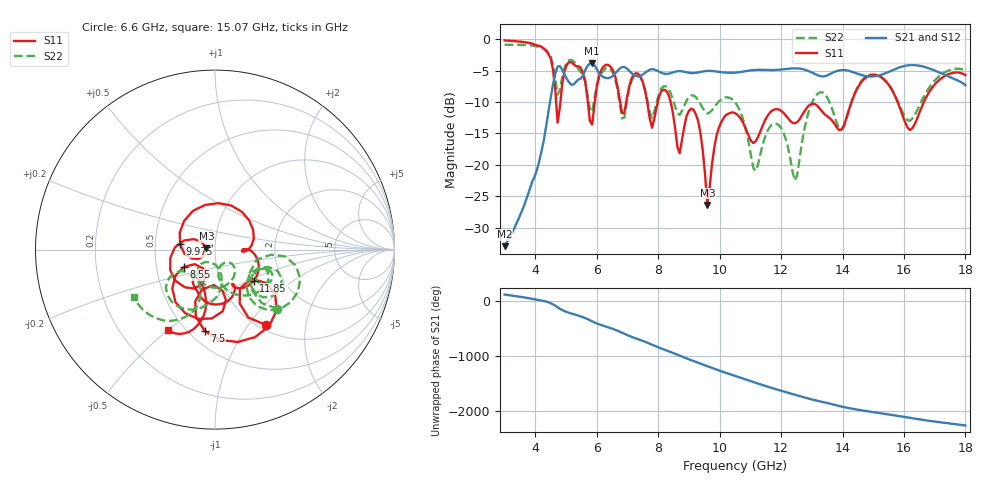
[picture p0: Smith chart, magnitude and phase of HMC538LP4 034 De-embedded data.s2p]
! Chelmsford, MA 01824
! http://www.hittite.com
! Tel: 978-250-3343
! Fax: 978-250-3373
! Device  :  HMC538LP4
! Description:  600 Analog Phase Shifter
! Frequency  :  6.0 GHz - 15.0 GHz
! Package  :  LP4  - 4x4 mm Quad Flatpack No-Lead (QFN) Plastic Package: 24 pin
! Ports  :  2 RF, 1 DC
!  Pin  3  = Rfin  = Port 1
!  Pin  16  = Rfout = Port 2
!  pin  21  = vCTL
! Voltages:  VCTL  = 0 to 5.0 Volts
! Currents :  Vb(V)  Vd(V)  Ib(mA)  Id(mA)
!  0.00  3.40  0.000000	0.470361
! Data:  The device was measured on evaluation board 111296-1.
!  Data was collected using a calibrated network analyzer.
!  The evaluation circuit board was modeled and simulated.This was use
!  to removed the evaluation board circuit from the measured data.
!  The reference plane is the center of the package pin.
! Misc:  Lot #
!Date Measured:  03 - 11 -2009
! Date:  03 - 17 -2009
! Note:
!  Hittite Microwave supplies this data as a sample of measured data at the
!  package pin for this package product.  Your particular data for this product
!  may vary.
!  Data was taken at 25 degrees C.
!  Hittite Microwave reserves the right to change this data at anytime.
# MHz S MA R 50
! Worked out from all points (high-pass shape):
!   201 points, 3 GHz to 18 GHz, reference 50 ohm
!   highest |S21| = -3.86 dB at 5.85 GHz (marker M1); lowest = -32.9 dB at 3 GHz (marker M2)
!   |S21| within 3 dB of the highest: 4.589 GHz to 5.097 GHz (508.1 MHz wide, 10.5 % of centre); 5.309 GHz to 17.87 GHz (12.56 GHz wide, 108 % of centre)
!   lowest |S11| = -26.4 dB at 9.6 GHz (marker M3), VSWR 1.10, Z = 45.5 + j0.618 ohm
!   |S11| at or under -10 dB: 7.641 GHz to 7.987 GHz (345.4 MHz wide, 4.42 % of centre); 8.406 GHz to 14.29 GHz (5.889 GHz wide, 51.9 % of centre); 15.79 GHz to 16.65 GHz (856.6 MHz wide, 5.28 % of centre)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
!   |S22| runs from -22.5 to -0.9 dB; largest |S21 - S12| = 0.0032
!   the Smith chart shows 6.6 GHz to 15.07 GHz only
!   S11 on the Smith chart (normalised r, x): 6.6 GHz: 1.08, -1.22; 7.5 GHz: 0.60, -0.68; 8.55 GHz: 0.70, -0.14; 9.975 GHz: 0.67, +0.04; 11.85 GHz: 1.43, -0.54; 15.07 GHz: 0.41, -0.50
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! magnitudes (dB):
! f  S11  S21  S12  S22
! 3 GHz  -0.2  -32.9  -32.9  -0.9
! 4.425 GHz  -2.4  -11.6  -11.6  -2.2
! 4.725 GHz  -13.3  -4.4  -4.4  -8.8
! 5.55 GHz  -5.3  -5.8  -5.8  -5.8
! 5.85 GHz  -13.6  -3.9  -3.9  -11.6
! 6.6 GHz  -5.9  -5.5  -5.5  -6.4
! 7.5 GHz  -6.8  -5.6  -5.6  -6.9
! 8.025 GHz  -9.2  -5.2  -5.2  -8.7
! 8.55 GHz  -14.1  -5.2  -5.2  -10.7
! 9.225 GHz  -11.9  -5.4  -5.4  -9.2
! 9.6 GHz  -26.4  -5.0  -5.0  -11.8
! 9.975 GHz  -14.1  -5.2  -5.2  -9.9
! 10.5 GHz  -11.8  -5.3  -5.3  -10.0
! 11.18 GHz  -16.2  -4.9  -4.9  -20.9
! 11.85 GHz  -11.1  -4.9  -4.9  -13.5
! 12.45 GHz  -13.4  -4.6  -4.6  -22.5
! 13.05 GHz  -10.3  -5.4  -5.4  -9.7
! 13.95 GHz  -14.4  -4.9  -4.9  -14.4
! 15.07 GHz  -5.7  -5.9  -5.9  -5.6
! 15.53 GHz  -7.4  -5.2  -5.2  -7.4
! 16.2 GHz  -14.5  -4.1  -4.1  -13.0
! 18 GHz  -5.7  -7.3  -7.3  -5.0
